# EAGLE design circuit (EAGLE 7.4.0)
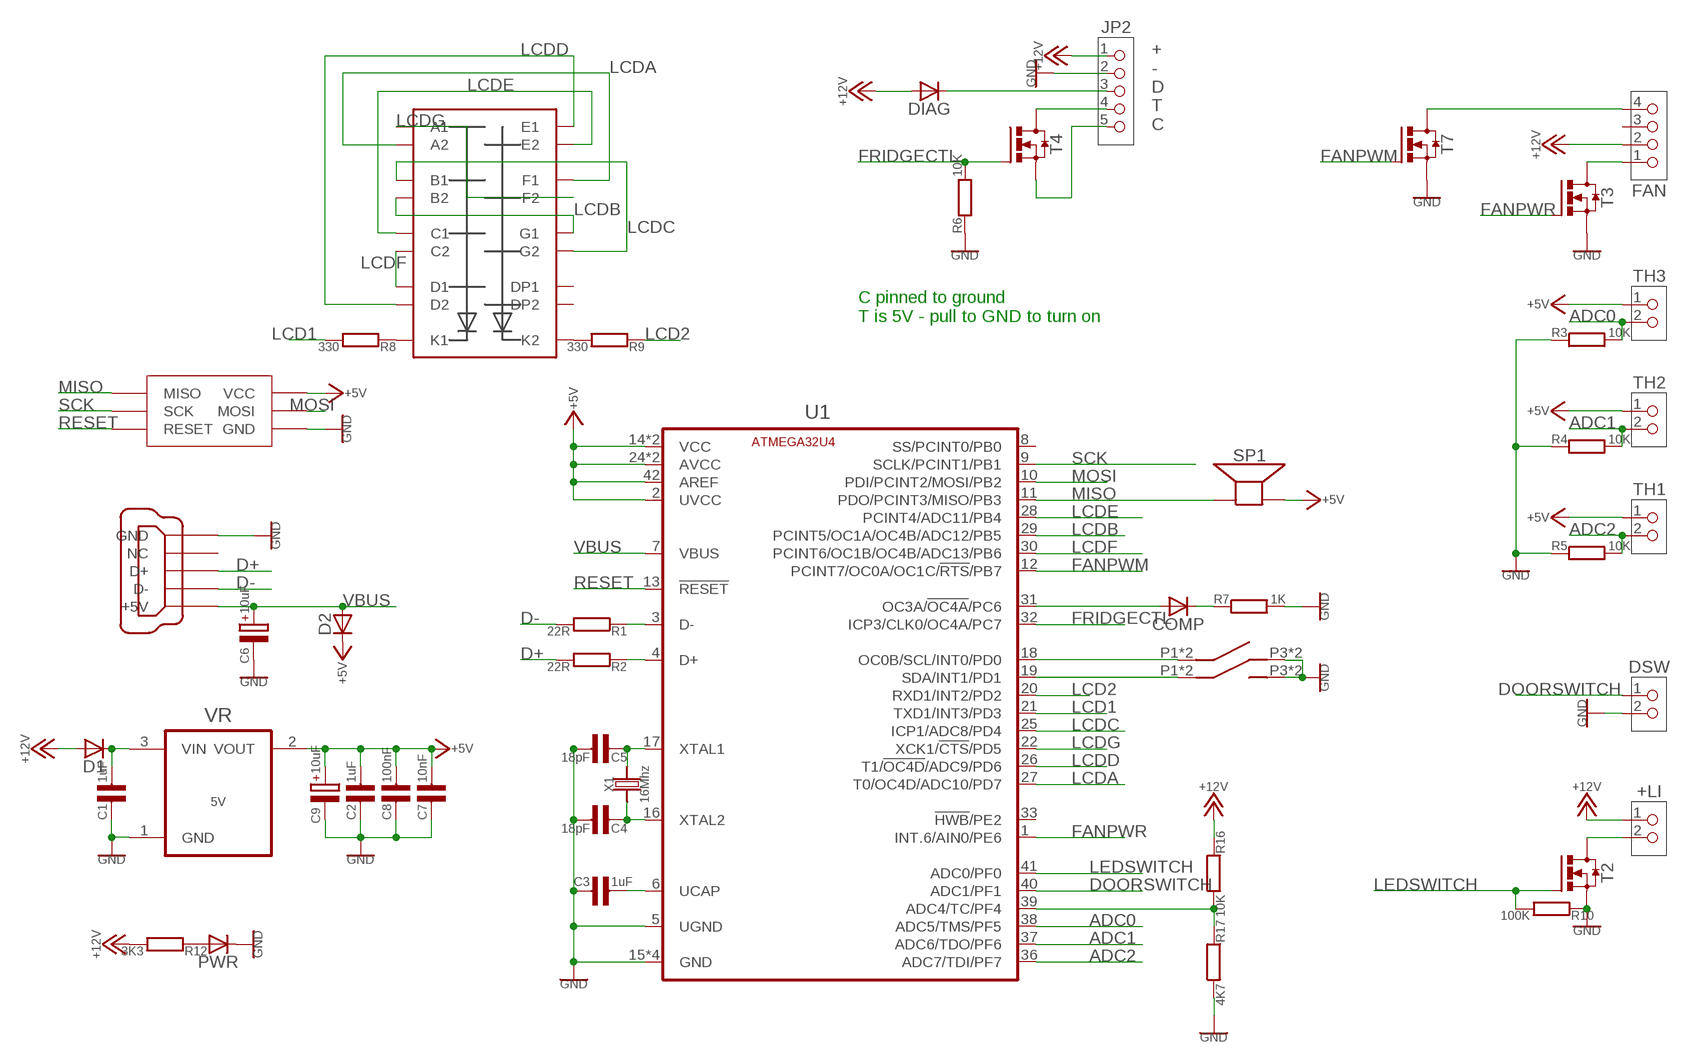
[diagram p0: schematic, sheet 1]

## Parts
+LI  PINHD-1X2  [1X02]
C1  1uF  C-EU0603  [0603]
C2  1uF  C-EU0603  [0603]
C3  1uF  C-EU0603  [0603]
C4  18pF  C-EU0603  [0603]
C5  18pF  C-EU0603  [0603]
C6  10uF  CAPACITOR-POLARISEDEIA3216  [EIA3216]
C7  10nF  C-EU0603  [0603]
C8  100nF  C-EU0603  [0603]
C9  10uF  CAPACITOR-POLARISEDEIA3216  [EIA3216]
COMP  DIODE0603  [0603-DIODE]
D1  DIODE0603  [0603-DIODE]
D2  DIODE0603  [0603-DIODE]
DIAG  DIODE0603  [0603-DIODE]
DSW  PINHD-1X2  [1X02]
FAN  PINHD-1X4MOLEX-FAN  [1X04-FAN]
JP2  PINHD-1X5  [1X05]
PWR  DIODE0603  [0603-DIODE]
R1  22R  R-EU0603  [0603]
R2  22R  R-EU0603  [0603]
R3  10K  R-EU0603  [0603]
R4  10K  R-EU0603  [0603]
R5  10K  R-EU0603  [0603]
R6  10K  R-EU0603  [0603]
R7  1K  R-EU0603  [0603]
R8  330  R-EU0603  [0603]
R9  330  R-EU0603  [0603]
R10  100K  R-EU0603  [0603]
R12  3K3  R-EU0603  [0603]
R16  10K  R-EU0603  [0603]
R17  4K7  R-EU0603  [0603]
SP1  PIEZOPIEZO-9MM  [PIEZO-9MM]
T2  BSS138  MOSFET-NCHSOT-23  [SOT23]
T3  AP2306  MOSFET-NCHSOT-23  [SOT23]
T4  AP2306  MOSFET-NCHSOT-23  [SOT23]
T7  AP2306  MOSFET-NCHSOT-23  [SOT23]
TH1  PINHD-1X2  [1X02]
TH2  PINHD-1X2  [1X02]
TH3  PINHD-1X2  [1X02]
U1  ATMEGA32U4  [QFN44]
U$1  KCDC04-107  [KCDC04-107]
U$2  SWITCH  [MULTICOMP-BUTTON]
U$3  SWITCH  [MULTICOMP-BUTTON]
U$4  AVRISPTAG-CONNECT  [TAG-CONNECT-2030NL]
USB  MINI-USB  [MINI-USB]
VR  5V  MCP1703SOT23  [SOT23]
X1  16Mhz  CRYSTAL3.2X2.5MM  [CRYSTAL-3.2X2.5MM]

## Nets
+5V: C2.1 C7.1 C8.1 C9.+ D2.2(K) SP1.P$2(-) TH1.1 TH2.1 TH3.1 U1.2(UVCC) U1.14(VCC) U1.24(AVCC) U1.34(VCC) U1.42(AREF) U1.44(AVCC) U$4.2(VCC) VR.2(VOUT)
+12V: +LI.1 D1.1(A) DIAG.1(A) FAN.2 JP2.1 R12.2 R16.1
ADC0: R3.2 TH3.2 U1.38(ADC5/TMS/PF5)
ADC1: R4.2 TH2.2 U1.37(ADC6/TDO/PF6)
ADC2: R5.2 TH1.2 U1.36(ADC7/TDI/PF7)
CNET: JP2.5 T4.2(S)
D+: R2.2 USB.3(D+)
D-: R1.2 USB.2(D-)
DIAGPIN: DIAG.2(K) JP2.3
DOORSWITCH: DSW.1 U1.40(ADC1/PF1)
FANPWM: T7.1(G) U1.12(PCINT7/OC0A/OC1C/!RTS!/PB7)
FANPWR: T3.1(G) U1.1(INT.6/AIN0/PE6)
FRIDGECTL: R6.2 T4.1(G) U1.32(ICP3/CLK0/OC4A/PC7)
GND: C1.2 C2.2 C3.2 C4.1 C5.1 C6.- C7.2 C8.2 C9.- DSW.2 JP2.2 PWR.2(K) R3.1 R4.1 R5.1 R6.1 R7.2 R10.1 R17.2 T2.2(S) T3.2(S) T7.2(S) U1.5(UGND) U1.15(GND) U1.23(GND) U1.35(GND) U1.43(GND) U$2.P3 U$2.P6 U$3.P3 U$3.P6 U$4.6(GND) USB.5(GND) VR.1(GND)
LCD1: R8.2 U1.21(TXD1/INT3/PD3)
LCD2: R9.1 U1.20(RXD1/INT2/PD2)
LCDA: U1.27(T0/OC4D/ADC10/PD7) U$1.P12(A2) U$1.P19(F1)
LCDB: U1.29(PCINT5/OC1A/OC4B/ADC12/PB5) U$1.P11(B2) U$1.P20(G1)
LCDC: U1.25(ICP1/ADC8/PD4) U$1.P15(G2) U$1.P16(B1)
LCDD: U1.26(T1/!OC4D!/ADC9/PD6) U$1.P1(E1) U$1.P7(D2)
LCDE: U1.28(PCINT4/ADC11/PB4) U$1.P4(C1) U$1.P6(E2)
LCDF: U1.30(PCINT6/OC1B/OC4B/ADC13/PB6) U$1.P2(D1) U$1.P9(C2)
LCDG: U1.22(XCK1/!CTS!/PD5) U$1.P14(F2) U$1.P17(A1)
LEDSWITCH: R10.2 T2.1(G) U1.41(ADC0/PF0)
MISO: SP1.P$1(+) U1.11(PDO/PCINT3/MISO/PB3) U$4.1(MISO)
MOSI: U1.10(PDI/PCINT2/MOSI/PB2) U$4.4(MOSI)
N$1: PWR.1(A) R12.1
N$2: COMP.2(K) R7.1
N$3: C3.1 U1.6(UCAP)
N$4: C5.2 U1.17(XTAL1) X1.3
N$5: C4.2 U1.16(XTAL2) X1.1
N$6: R2.1 U1.4(D+)
N$7: R1.1 U1.3(D-)
N$9: R8.1 U$1.P3(K1) U$1.P18(K1)
N$10: FAN.1 T3.3(D)
N$11: C1.1 D1.2(K) VR.3(VIN)
N$12: R9.2 U$1.P8(K2) U$1.P13(K2)
N$13: COMP.1(A) U1.31(OC3A/!OC4A!/PC6)
N$14: R16.2 R17.1 U1.39(ADC4/TC/PF4)
N$15: U1.18(OC0B/SCL/INT0/PD0) U$2.P1 U$2.P4
N$16: U1.19(SDA/INT1/PD1) U$3.P1 U$3.P4
RESET: U1.13(!RESET!) U$4.5(RESET)
SCK: U1.9(SCLK/PCINT1/PB1) U$4.3(SCK)
SWITCH2: +LI.2 T2.3(D)
TNET: JP2.4 T4.3(D)
VBUS: C6.+ D2.1(A) U1.7(VBUS) USB.1(+5V)
Z: FAN.4 T7.3(D)
Unconnected: FAN.3 U1.8(SS/PCINT0/PB0) U1.33(!HWB!/PE2) U$1.P5(DP1) U$1.P10(DP2) USB.4(NC)

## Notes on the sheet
- +
  -
  D
  T
  C
- C pinned to ground
  T is 5V - pull to GND to turn on

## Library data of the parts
+LI DSW TH1-TH3 = MikesParts:PINHD-1X2: PIN HEADER
C1-C5 C7 C8 = MikesParts:C-EU
C6 C9 = MikesParts:CAPACITOR-POLARISED: Polarised Capacitor
COMP D1 D2 DIAG PWR = MikesParts:DIODE
FAN = MikesParts:PINHD-1X4: PIN HEADER
JP2 = MikesParts:PINHD-1X5: PIN HEADER
R1-R10 R12 R16 R17 = MikesParts:R-EU
SP1 = MikesParts:PIEZO
T2-T4 T7 = MikesParts:MOSFET-NCH: MOSFET N-Channel, eg BSS138, BUK7Y13, FDN335N
U1 = MikesParts:ATMEGA32U4
U$1 = MikesParts:KCDC04-107: Kingbright 2 digit 7 segment display (common cathode)
U$2 U$3 = MikesParts:SWITCH
U$4 = MikesParts:AVRISP
USB = MikesParts:MINI-USB: MINI USB-B Conector Source: www.cypressindustries.com
VR = MikesParts:MCP1703: IC REG LDO 250MA: 2V5, 3V3, 5V0
X1 = MikesParts:CRYSTAL

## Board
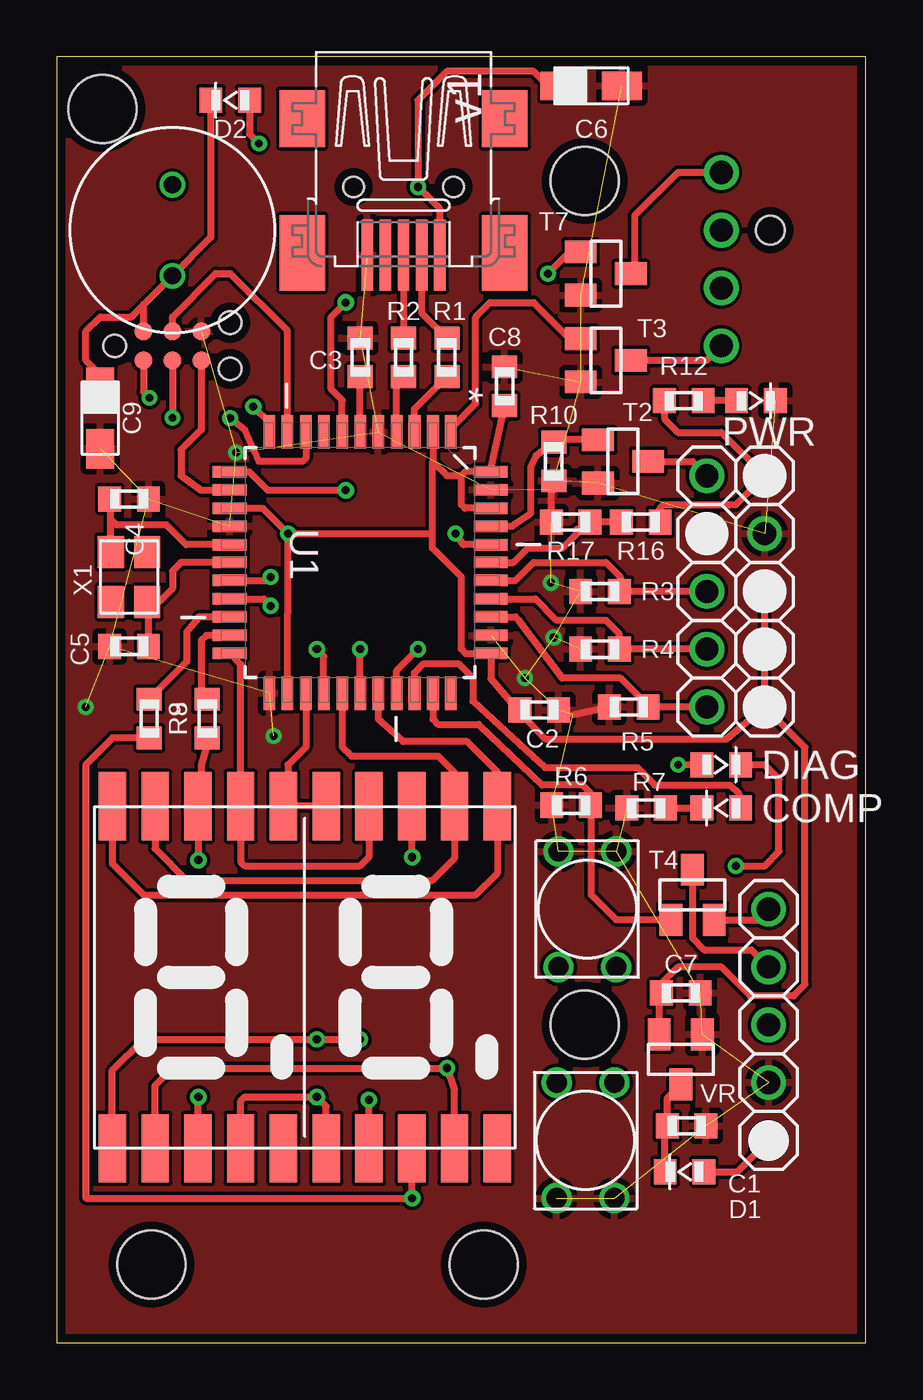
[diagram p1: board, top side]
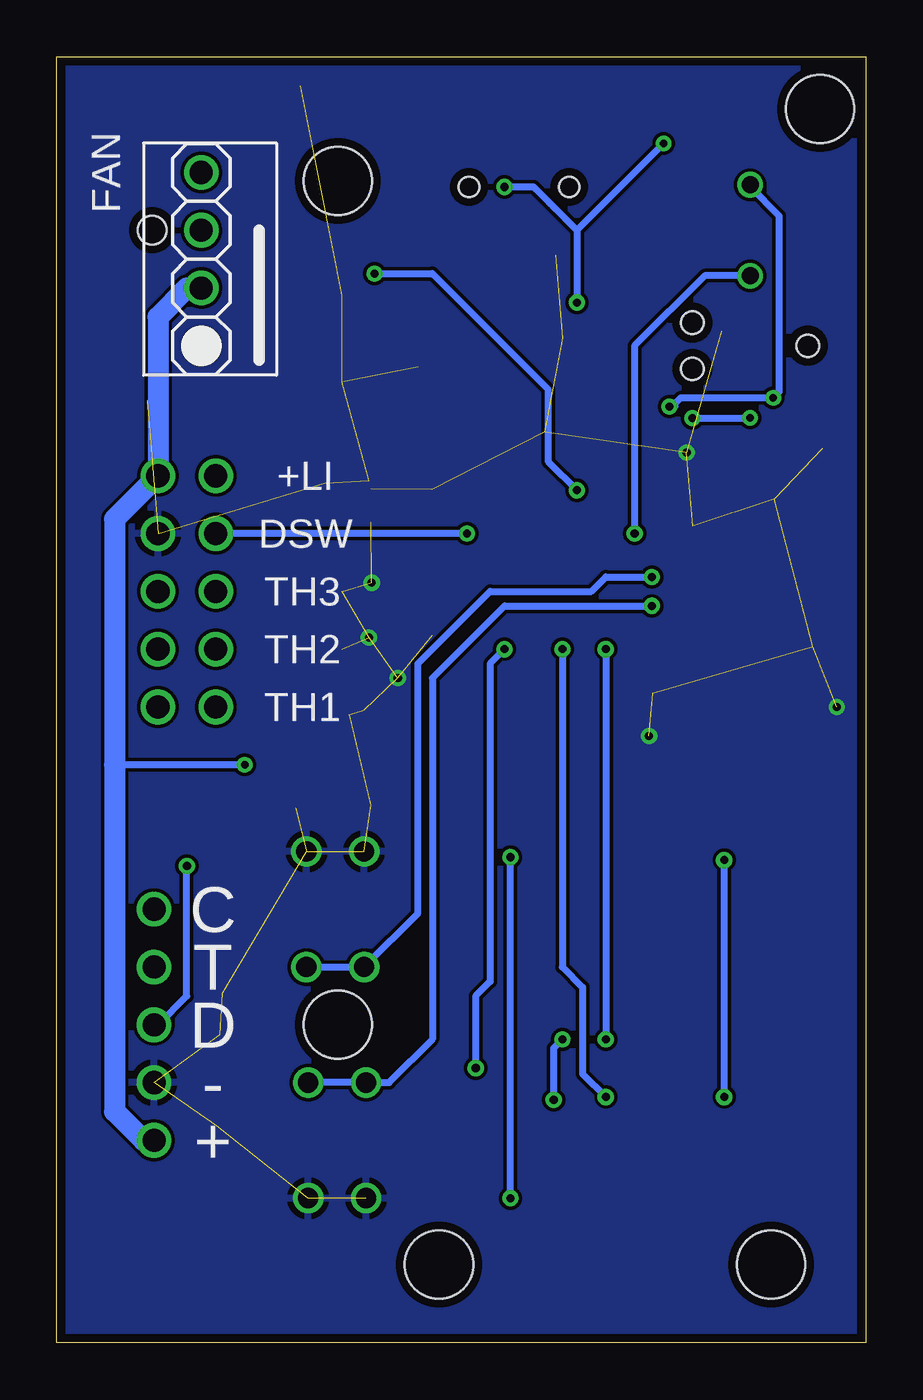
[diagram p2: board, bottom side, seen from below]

Size 35.56 x 56.52 mm. Coordinates in mm from the lower left corner, seen from the top.
Outline: 0,56.52 0,0 35.56,0 35.56,56.52 0,56.52
Copper layers (1*16): Top 0.0356mm / dielectric 1.5011mm / Bottom 0.0356mm
Design rules "LaenPCBOrder": minimum track width 6mil, minimum drill 13mil, track to track 6mil, track to pad 6mil, pad to pad 6mil, via to via 6mil, smd to smd 6mil, copper to edge 15mil, drill to drill 6mil, minimum pad ring 7mil, minimum via ring 7mil, stop-mask expansion 4mil, vias tented up to drill 0mil, thermal gap 10mil
Holes 3 mm at 23.21,13.97 23.2,51.05 2,54.23 4.16,3.43 18.76,3.43

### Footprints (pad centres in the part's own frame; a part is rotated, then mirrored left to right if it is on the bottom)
1X02 = drill 1.016: 1 -1.27,0; 2 1.27,0
0603 = smd 1 x 1.1: 1 -0.85,0; 2 0.85,0
EIA3216 = smd 1.75 x 1.25: + -1.35,0; - 1.35,0
0603-DIODE = smd 1 x 1.1: 1 -0.85,0; 2 0.85,0
1X04-FAN = drill 1.016: 1 3.81,0; 2 1.27,0; 3 -1.27,0; 4 -3.81,0 | hole 1.25: -1.27,-2.16
1X05 = drill 1.016: 1 -5.08,0; 2 -2.54,0; 3 0,0; 4 2.54,0; 5 5.08,0
PIEZO-9MM = drill 0.75: P$1 -2,0; P$2 2,0
SOT23 = smd 1 x 1.4: 1 -0.95,-1.1; 2 0.95,-1.1; 3 0,1.1
QFN44 = smd 1.473 x 0.508: 1 -5.74,3.988; 2 -5.74,3.2; 3 -5.74,2.388; 4 -5.74,1.6; 5 -5.74,0.787; 6 -5.74,0; 7 -5.74,-0.787; 8 -5.74,-1.6; 9 -5.74,-2.388; 10 -5.74,-3.2; 11 -5.74,-3.988; 23 5.74,-3.988; 24 5.74,-3.2; 25 5.74,-2.388; 26 5.74,-1.6; 27 5.74,-0.787; 28 5.74,0; 29 5.74,0.787; 30 5.74,1.6; 31 5.74,2.388; 32 5.74,3.2; 33 5.74,3.988 | smd 0.508 x 1.473: 12 -3.988,-5.74; 13 -3.2,-5.74; 14 -2.388,-5.74; 15 -1.6,-5.74; 16 -0.787,-5.74; 17 0,-5.74; 18 0.787,-5.74; 19 1.6,-5.74; 20 2.388,-5.74; 21 3.2,-5.74; 22 3.988,-5.74; 34 3.988,5.74; 35 3.2,5.74; 36 2.388,5.74; 37 1.6,5.74; 38 0.787,5.74; 39 0,5.74; 40 -0.787,5.74; 41 -1.6,5.74; 42 -2.388,5.74; 43 -3.2,5.74; 44 -3.988,5.74
KCDC04-107 = smd 1.2 x 3: P1 -8.46,-7.52; P2 -6.58,-7.52; P3 -4.7,-7.52; P4 -2.82,-7.52; P5 -0.94,-7.52; P6 0.94,-7.52; P7 2.82,-7.52; P8 4.7,-7.52; P9 6.58,-7.52; P10 8.46,-7.52; P11 8.46,7.52; P12 6.58,7.52; P13 4.7,7.52; P14 2.82,7.52; P15 0.94,7.52; P16 -0.94,7.52; P17 -2.82,7.52; P18 -4.7,7.52; P19 -6.58,7.52; P20 -8.46,7.52
MULTICOMP-BUTTON = drill 0.889: P1 -1.27,2.54; P3 -1.27,-2.54; P4 1.27,2.54; P6 1.27,-2.54
TAG-CONNECT-2030NL = smd 0.787 x 0.787: 1 -1.27,-0.635; 2 -1.27,0.635; 3 0,-0.635; 4 0,0.635; 5 1.27,-0.635; 6 1.27,0.635 | hole 0.991: -2.54,0; 2.54,1.016; 2.54,-1.016
MINI-USB = smd 3.1 x 0.5: 1 3,1.6; 2 3,0.8; 3 3,0; 4 3,-0.8; 5 3,-1.6 | smd 2.5 x 2: M1 -3,-4.45; M2 -3,4.45 | smd 3.3 x 2: M3 2.9,4.45; M4 2.9,-4.45 | hole 0.9: 0,2.2; 0,-2.2
CRYSTAL-3.2X2.5MM = smd 1.4 x 1.15: 1 -1.1,-0.8; 2 1.1,-0.8; 3 1.1,0.8; 4 -1.1,0.8

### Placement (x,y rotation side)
+LI  29.84,38.1 180 top
C1  27.69,9.53 0 top
C2  21.21,27.81 0 top
C3  13.34,43.31 90 top
C4  3.17,37.08 180 top
C5  3.17,30.61 0 top
C6  23.5,55.24 0 top
C7  27.43,15.37 0 top
C8  19.68,42.04 90 top
C9  1.91,40.64 270 top
COMP  29.21,23.5 180 top
D1  27.59,7.51 180 top
D2  7.62,54.61 180 top
DIAG  29.21,25.4 0 top
DSW  29.84,35.56 0 top
FAN  29.21,47.62 270 bottom
JP2  31.29,13.97 90 top
PWR  30.73,41.4 0 top
R1  17.14,43.31 90 top
R2  15.24,43.31 90 top
R3  23.88,33.02 0 top
R4  23.88,30.48 0 top
R5  25.15,27.94 0 top
R6  22.61,23.62 0 top
R7  25.91,23.5 180 top
R8  6.6,27.43 90 top
R9  4.06,27.43 270 top
R10  21.84,38.73 90 top
R12  27.56,41.4 180 top
R16  25.67,36.07 180 top
R17  22.59,36.07 180 top
SP1  5.08,48.9 270 top
T2  24.89,38.73 270 top
T3  24.13,43.18 270 top
T4  27.94,19.68 0 top
T7  24.13,46.99 270 top
TH1  29.84,27.94 180 top
TH2  29.84,30.48 180 top
TH3  29.84,33.02 180 top
U1  13.34,34.29 270 top
U$1  10.9,16.06 0 top
U$2  23.32,19.05 180 top
U$3  23.24,8.89 0 top
U$4  5.08,43.81 0 top
USB  15.24,50.8 270 top
VR  27.43,12.45 180 top
X1  3.17,33.66 270 top

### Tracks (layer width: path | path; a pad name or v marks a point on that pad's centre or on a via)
+5V  (via drill 0.36)
  Top 0.305: U1.42 17.93,36.68 17.78,36.83 17.78,38.1 | U1.2 16.54,38.71 | 16.54,38.71 17.14,38.1 17.78,38.1 | 17.78,38.1 17.96,38.28 U1.44 19.05,38.3 C8.1 | 16.51,35.56 16.51,34.92 17.78,33.66 17.78,30.48 17.98,30.28 19.05,30.28 U1.34 19.07,29.18 20.36,27.7 | 16.51,35.56 16.51,38.68 16.54,38.71 | U1.24 v10.16,35.56 | v10.16,35.56 9.04,36.68 U1.14 | v10.16,35.56 16.51,35.56 | TH1.1 TH2.1 TH3.1 | 20.36,27.7 21.46,26.54 29.46,26.54 TH1.1 | TH1.1 32.89,26.16 32.89,15.75 32.38,15.24 30.48,15.24 29.21,16.51 27.3,16.51 26.58,15.79 C7.1 26.48,15.27 VR.2 | C2.1 20.09,27.94 20.36,27.7 | U$4.2 3.81,45.62 | 3.81,45.62 SP1.P$2 6.77,48.59 D2.2 | C9.+ 1.91,42.55 1.27,43.18 1.27,44.45 1.91,45.09 3.27,45.09 3.81,45.62
  Bottom 0.305: SP1.P$2 7.08,46.9 10.16,43.81 v10.16,35.56
+12V  (via drill 0.33)
  Top 0.305: R16.1 26.52,36.68 26.67,36.83 29.84,36.83 +LI.1 29.21,40.01 27.3,40.01 26.71,40.6 R12.2 | D1.1 29.91,7.51 JP2.1 | DIAG.1 v27.3,25.4
  Bottom 0.305: v27.3,25.4 33.02,25.4
  Bottom 0.914: FAN.2 29.84,46.35 31.11,45.09 +LI.1 33.02,36.2 33.02,25.4 33.02,10.16 31.75,8.89 JP2.1
ADC0
  Top 0.305: TH3.2 R3.2 24.77,33.06 24.77,33.66 24.13,34.29 20.95,34.29 20.17,33.5 U1.38
ADC1
  Top 0.305: TH2.2 R4.2 24.73,31.15 24.13,31.75 21.97,31.75 21.03,32.69 U1.37
ADC2
  Top 0.305: TH1.2 R5.2 26,27.98 24.77,29.21 22.23,29.21 20.32,31.75 20.17,31.9 U1.36
CNET
  Top 0.305: JP2.5 30.82,18.59 T4.2
D+
  Top 0.305: USB.3 R2.2
D-
  Top 0.305: USB.2 16.04,45.26 R1.2
DIAGPIN  (via drill 0.36)
  Top 0.305: v29.84,20.95 31.11,20.95 31.75,21.59 31.75,24.77 31.11,25.4 DIAG.2
  Bottom 0.305: v29.84,20.95 29.84,15.24 31.11,13.97 JP2.3
DOORSWITCH  (via drill 0.36)
  Top 0.305: U1.40 17.88,35.08 v17.53,35.56
  Bottom 0.305: v17.53,35.56 DSW.1
FANPWM  (via drill 0.36)
  Top 0.305: T7.1 22.54,47.94 v21.59,46.99 | U1.12 8.46,38.28 9.27,37.47 v12.7,37.47
  Bottom 0.305: v21.59,46.99 19.05,46.99 13.97,41.91 13.97,38.73 v12.7,37.47
FANPWR
  Top 0.305: U1.1 17.32,40.18 18.41,41.27 18.41,45.09 19.05,45.72 20.95,45.72 22.55,44.13 T3.1
FRIDGECTL
  Top 0.305: U1.32 16.54,27.41 16.76,27.18 18.54,27.18 21.34,24.51 23.11,24.51 23.46,24.17 R6.2 23.5,23.58 23.5,19.68 24.59,18.59 T4.1
GND  (via drill 0.36)  (38 unrouted)
  Top 0.305: 22.69,27.6 R5.1 | R17.2 21.74,37.53 R10.1
  other vias: 1.27,27.94 9.53,26.67 21.72,33.4 21.84,30.99 20.57,29.21 7.87,39.12
  pour Top: 0,56.52 36.2,56.52 36.2,0 0,0
  pour Bottom: 0,56.52 36.2,56.52 36.2,0 0,0
LCD1
  Top 0.305: U1.21 6.58,31.09 6.35,30.86 6.35,28.54 R8.2
LCD2
  Top 0.305: U1.20 6.25,31.9 5.71,31.24 5.71,29.93 R9.1
LCDA
  Top 0.305: U$1.P19 4.32,21.71 5.71,20.32 16.51,20.32 17.48,21.29 U$1.P12 17.48,25.07 16.76,25.78 12.95,25.78 12.55,26.19 U1.27
LCDB
  Top 0.305: U$1.P20 2.44,21.05 3.81,19.68 18.41,19.68 19.36,20.63 U$1.P11 19.36,25.09 18.03,26.42 15.24,26.42 14.12,27.41 U1.29
LCDC
  Top 0.305: U$1.P15 U$1.P16 10.16,23.78 10.16,25.4 10.95,26.19 U1.25
LCDD  (via drill 0.36)
  Top 0.305: U$1.P1 2.44,11.96 3.81,13.34 v11.43,13.34 v13.34,13.34 | U$1.P7 v13.72,10.66 v13.72,10.67 | U1.26 11.73,30.18 v11.43,30.48
  Bottom 0.305: v13.72,10.67 13.72,12.95 v13.34,13.34 | v11.43,30.48 v11.43,13.34
LCDE  (via drill 0.36)
  Top 0.305: U$1.P4 8.08,10.62 8.26,10.79 v11.43,10.79 11.84,10.38 U$1.P6 | U1.28 v13.34,30.48
  Bottom 0.305: v13.34,30.48 13.34,16.51 12.45,15.62 12.45,11.81 v11.43,10.79
LCDF  (via drill 0.36)
  Top 0.305: U$1.P2 4.32,11.3 5.08,12.06 v17.14,12.06 17.48,11.1 U$1.P9 | U1.30 14.94,29.54 v15.88,30.48
  Bottom 0.305: v15.88,30.48 16.51,29.84 16.51,15.88 17.14,15.24 v17.14,12.06
LCDG
  Top 0.305: U$1.P14 13.72,21.34 13.34,20.95 8.26,20.95 8.08,21.13 U$1.P17 8.08,29.82 U1.22
LEDSWITCH
  Top 0.305: T2.1 21.94,39.69 R10.2 21.04,38.95 20.83,38.48 20.83,36.45 20.02,35.89 U1.41
MISO  (via drill 0.33, 0.36)
  Top 0.305: U1.11 9.35,40.44 v8.64,41.15 | U$4.1 3.81,41.78 v4.06,41.53
  Bottom 0.305: v8.64,41.15 8.38,41.15 8.38,41.27 8.13,41.53 v4.06,41.53 3.81,41.78 3.81,49.53 5.08,50.8 SP1.P$1
MOSI
  Top 0.305: U$4.4 5.08,45.09 6.99,46.99 7.62,46.99 10.13,44.48 U1.10
N$1
  Top 0.305: PWR.1 R12.1
N$2
  Top 0.305: R7.1 COMP.2
N$3
  Top 0.305: U1.6 C3.1
N$4
  Top 0.305: U1.17 5.46,34.29 5.08,33.91 5.08,33.15 4.49,32.55 X1.3 4.03,32.51 C5.2
N$5
  Top 0.305: X1.1 2.38,36.2 | 2.38,36.2 2.38,37.03 C4.2 | U1.16 5.69,35.08 4.83,35.94 2.63,35.94 2.38,36.2
N$6
  Top 0.305: U1.4 14.94,42.15 R2.1
N$7
  Top 0.305: U1.3 15.72,41.03 R1.1
N$9  (via drill 0.36)
  Top 0.305: U$1.P3 6.2,10.18 v6.22,10.79 | v6.22,21.21 6.2,21.23 U$1.P18 6.35,23.73 6.35,25.4 6.6,26.29 R8.1
  Bottom 0.305: v6.22,10.79 v6.22,21.21
N$10
  Top 0.305: T3.3 28.57,43.18 FAN.1
N$11
  Top 0.305: D1.2 26.74,9.43 C1.1 26.84,10.75 VR.3
N$12  (via drill 0.36)
  Top 0.305: U$1.P8 15.6,6.37 v15.62,6.35 1.27,6.35 1.27,25.4 2.45,26.58 R9.2 | v15.62,21.34 15.62,23.56 U$1.P13
  Bottom 0.305: v15.62,6.35 v15.62,21.34
N$13
  Top 0.305: U1.31 15.72,29.44 16.13,29.84 17.65,29.84 18.29,29.21 18.29,28.19 21.46,25.27 25.53,25.27 26.29,24.51 29.59,24.51 29.97,24.13 29.97,23.58 COMP.1
N$14
  Top 0.305: R16.2 R17.1 22.86,35.74 22.86,35.56 22.23,34.92 20.7,34.92 20.07,34.29 U1.39
N$15  (via drill 0.36)
  Top 0.305: U1.18 9.25,33.5 v9.4,33.66
  Bottom 0.305: U$2.P1 U$2.P4 19.68,18.88 19.68,29.84 16.51,33.02 12.06,33.02 11.43,33.66 v9.4,33.66
N$16  (via drill 0.36)
  Top 0.305: U1.19 9.09,32.69 v9.4,32.38
  Bottom 0.305: U$3.P4 U$3.P1 20.95,11.43 19.05,13.34 19.05,29.21 15.88,32.38 v9.4,32.38
RESET
  Top 0.305: U1.13 7.57,37.47 6.35,37.47 5.46,38.1 5.46,39.24 6.35,40.13 U$4.5
SCK  (via drill 0.33, 0.36)
  Top 0.305: U1.9 10.95,38.89 10.79,38.73 8.89,38.73 8.26,40.13 v7.62,40.64 | U$4.3 v5.08,40.64
  Bottom 0.305: v7.62,40.64 v5.08,40.64
SWITCH2
  Top 0.305: T2.3 27.94,38.73 +LI.2
TNET
  Top 0.305: T4.3 27.94,17.78 28.45,17.27 30.53,17.27 JP2.4
VBUS  (via drill 0.33, 0.36)
  Top 0.305: USB.1 16.84,49.84 v15.88,50.8 15.88,54.61 17.14,55.88 20.95,55.88 21.59,55.24 C6.+ | U1.7 12.55,41.43 12.06,41.91 12.06,45.09 v12.7,45.72 | D2.1 8.47,53.12 v8.89,52.7
  Bottom 0.305: v15.88,50.8 14.61,50.8 12.7,48.9 | 12.7,48.9 v12.7,45.72 | 12.7,48.9 v8.89,52.7
Z
  Top 0.305: FAN.4 27.3,51.44 25.4,49.53 25.4,47.16 T7.3

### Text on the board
tNames: v1
bNames: C | T | D | - | +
